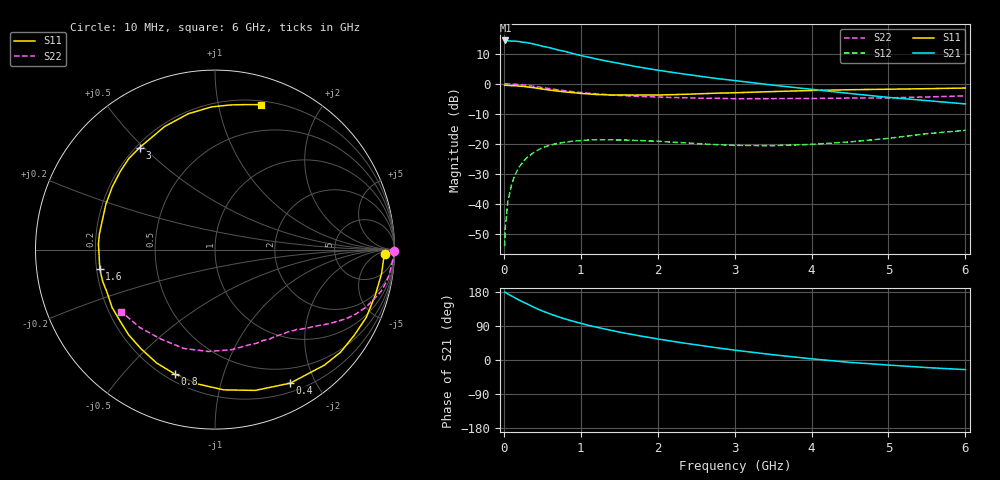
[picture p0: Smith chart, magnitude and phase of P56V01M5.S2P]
! SIEMENS Small Signal Semiconductors
! BFP183
! Si NPN RF Bipolar Junction Transistor in SOT143
! VCE = 6 V  IC = 1.5 mA
! Common Emitter S-Parameters:  March  1996
# GHz  S  MA  R  50
!  f  S11  S21  S12  S22
! GHz  MAG  ANG  MAG  ANG  MAG  ANG  MAG  ANG
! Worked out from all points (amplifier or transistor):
!   36 points, 10 MHz to 6 GHz, reference 50 ohm
!   highest |S21| = 14.4 dB at 20 MHz (marker M1)
!   |S21| within 3 dB of that: start of sweep to 682.3 MHz
!   unconditionally stable (mu >= 1): 2.321 GHz to 5.901 GHz
!   at 250 MHz: K = 0.10, MSG = 19.9 dB, |S12| = -25.9 dB
!   at 1.4 GHz: K = 0.60, MSG = 12.9 dB, |S12| = -18.6 dB
!   at 6 GHz: K = 0.98, MSG = 4.4 dB, |S12| = -15.5 dB
!   S11 on the Smith chart (normalised r, x): 10 MHz: 29, -14; 400 MHz: 0.30, -1.67; 800 MHz: 0.24, -0.70; 1.6 GHz: 0.21, -0.08; 3 GHz: 0.21, +0.49; 6 GHz: 0.23, +1.34
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0.01  0.9454 -1.6  5.169 179.2  0.002 85.8  0.9999 -0.6
0.02  0.9408 -3.3  5.232 178.4  0.0041 86.2  0.9982 -1.2
0.05  0.9378 -8.1  5.19 174.5  0.0107 89.1  0.9936 -2.9
0.1  0.9287 -15.8  5.091 169.1  0.021 79.8  0.9855 -5.7
0.15  0.9234 -24.2  5.099 163.5  0.0316 76.0  0.9798 -8.7
0.25  0.9034 -39.3  4.883 152.9  0.0505 67.4  0.9546 -14.0
0.3  0.8864 -46.6  4.823 148.3  0.059 63.3  0.9355 -16.3
0.4  0.854 -60.6  4.527 138.2  0.0739 55.4  0.9011 -20.8
0.5  0.8161 -74.0  4.201 129.5  0.0861 48.4  0.8634 -24.5
0.6  0.7829 -86.5  3.955 121.7  0.0954 42.2  0.8271 -27.7
0.8  0.7284 -108.0  3.427 108.1  0.1069 32.4  0.7624 -32.6
0.9  0.7107 -117.2  3.166 102.3  0.1113 28.1  0.7358 -34.7
1.1  0.6762 -135.3  2.764 91.3  0.1162 21.4  0.6945 -38.1
1.4  0.6474 -157.8  2.297 78.0  0.1171 13.5  0.6525 -42.8
1.6  0.6508 -170.6  2.06 69.9  0.1158 10.1  0.6303 -45.5
1.8  0.6502 177.3  1.849 62.4  0.1134 7.5  0.6123 -48.5
2.2  0.6585 157.4  1.538 49.0  0.1066 4.3  0.589 -55.0
3  0.707 126.5  1.128 26.0  0.0944 6.3  0.564 -70.1
3.5  0.7408 112.3  0.947 13.9  0.0934 11.8  0.5653 -80.8
4.5  0.7949 91.5  0.688 -6.3  0.1081 22.7  0.5774 -107.4
5.5  0.827 77.7  0.524 -20.0  0.148 25.7  0.6031 -133.9
6  0.8475 72.3  0.461 -25.4  0.1679 22.8  0.6264 -146.5
